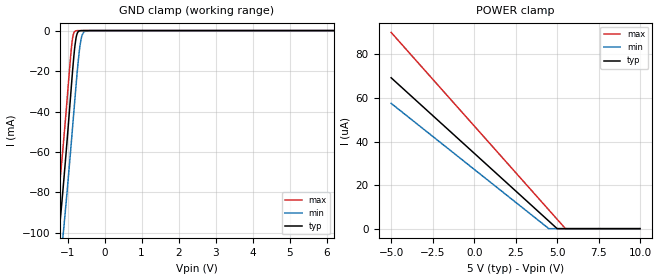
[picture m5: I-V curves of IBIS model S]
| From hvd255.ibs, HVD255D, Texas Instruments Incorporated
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[Model]   S
Model_type   Input
Vinl = .8
Vinh = 2
|   typ   min   max
|   (nom PVT)   (slow PVT)   (fast PVT)
C_comp   3.6778e-13   3.5291e-13   3.9050e-13
[Voltage Range]   5   4.5   5.5
[Temperature Range]   27   125   -40
[Power Clamp Reference]   5   4.5   5.5
[GND Clamp Reference]   -0   -0   -0
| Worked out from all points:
|   GND clamp passes 1 mA (typ) near -0.73 V on its own axis
[GND Clamp]
|   Voltage   I(typ)   I(min)   I(max)
-5V       -570.9mA   -586.3mA   -524.8mA
-1.52V    -152.4mA   -171.3mA   -129.5mA
-1.25V    -104mA     -125.3mA   -82.98mA
-1.175V   -89.21mA   -111.5mA   -68.54mA
-1.1V     -73.64mA   -97.17mA   -53.2mA
-890mV    -25.88mA   -53.52mA   -7.604mA
-845mV    -15.82mA   -43.57mA   -1.977mA
-770mV    -3.606mA   -27.02mA   -95.72uA
-680mV    -177.9uA   -9.849mA   -20.15uA
-620mV    -24.13uA   -3.133mA   -12.35uA
-410mV    -2.813uA   -12.82uA   -3.509uA
9.985V    0A         0A         0A
[POWER Clamp]
|   Voltage   I(typ)   I(min)   I(max)
-5V       69.31uA    57.56uA    90.13uA
4.48V     3.57uA     79.77nA    8.723uA
4.99V     30.25nA    0A         4.345uA
5.485V    0A         0A         91.39nA
9.985V    0A         0A         0A
